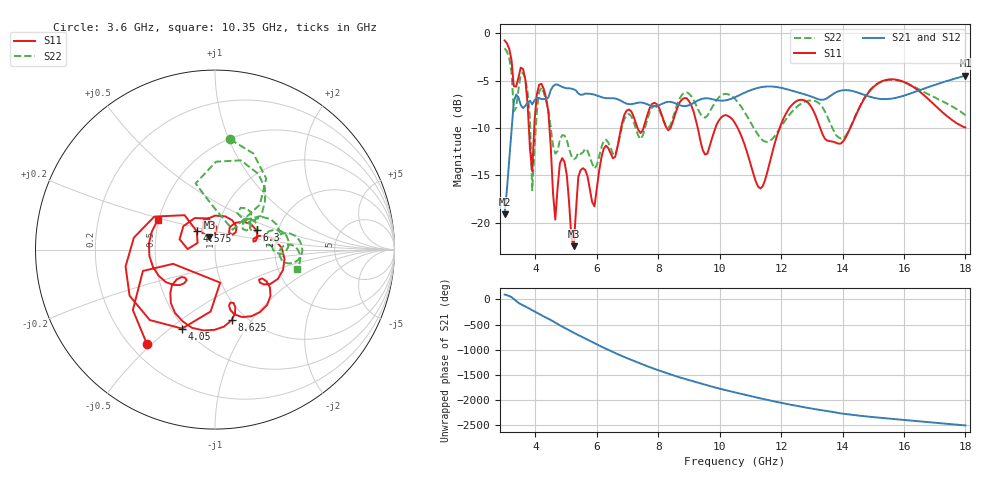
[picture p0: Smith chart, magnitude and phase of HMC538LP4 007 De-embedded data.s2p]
! Chelmsford, MA 01824
! http://www.hittite.com
! Tel: 978-250-3343
! Fax: 978-250-3373
! Device  :  HMC538LP4
! Description:  600 Analog Phase Shifter
! Frequency  :  6.0 GHz - 15.0 GHz
! Package  :  LP4  - 4x4 mm Quad Flatpack No-Lead (QFN) Plastic Package: 24 pin
! Ports  :  2 RF, 1 DC
!  Pin  3  = Rfin  = Port 1
!  Pin  16  = Rfout = Port 2
!  pin  21  = vCTL
! Voltages:  VCTL  = 0 to 5.0 Volts
! Currents :  Vb(V)  Vd(V)  Ib(mA)  Id(mA)
!  0.00  0.70  0.000000	0.484032
! Data:  The device was measured on evaluation board 111296-1.
!  Data was collected using a calibrated network analyzer.
!  The evaluation circuit board was modeled and simulated.This was use
!  to removed the evaluation board circuit from the measured data.
!  The reference plane is the center of the package pin.
! Misc:  Lot #
!Date Measured:  03 - 11 -2009
! Date:  03 - 17 -2009
! Note:
!  Hittite Microwave supplies this data as a sample of measured data at the
!  package pin for this package product.  Your particular data for this product
!  may vary.
!  Data was taken at 25 degrees C.
!  Hittite Microwave reserves the right to change this data at anytime.
# MHz S MA R 50
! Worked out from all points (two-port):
!   201 points, 3 GHz to 18 GHz, reference 50 ohm
!   highest |S21| = -4.46 dB at 18 GHz (marker M1); lowest = -19.1 dB at 3 GHz (marker M2)
!   |S21| within 3 dB of the highest: 3.909 GHz to 7.012 GHz (3.103 GHz wide, 56.8 % of centre); 9.097 GHz to end of sweep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
!   lowest |S11| = -22.5 dB at 5.25 GHz (marker M3), VSWR 1.16, Z = 46.6 + j6.4 ohm
!   |S11| at or under -10 dB: 4.461 GHz to 6.792 GHz (2.331 GHz wide, 41.4 % of centre); 10.59 GHz to 11.96 GHz (1.369 GHz wide, 12.1 % of centre); 13.27 GHz to 14.25 GHz (985.1 MHz wide, 7.16 % of centre)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
!   |S22| runs from -16.6 to -1.6 dB; largest |S21 - S12| = 0.0017
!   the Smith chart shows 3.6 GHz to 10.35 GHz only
!   S11 on the Smith chart (normalised r, x): 3.6 GHz: 0.27, -0.48; 4.05 GHz: 0.48, -0.55; 4.575 GHz: 0.80, +0.17; 6.3 GHz: 1.55, +0.36; 8.625 GHz: 0.85, -0.80; 10.35 GHz: 0.49, +0.19
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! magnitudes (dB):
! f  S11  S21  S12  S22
! 3 GHz  -0.8  -19.1  -19.1  -1.6
! 3.3 GHz  -5.6  -7.2  -7.2  -8.2
! 3.6 GHz  -3.8  -7.9  -7.9  -4.2
! 3.825 GHz  -12.2  -7.1  -7.1  -9.0
! 3.9 GHz  -14.6  -7.5  -7.5  -16.6
! 4.05 GHz  -6.4  -6.8  -6.8  -8.3
! 4.35 GHz  -6.8  -6.9  -6.9  -7.1
! 4.575 GHz  -16.9  -5.6  -5.6  -11.9
! 4.95 GHz  -13.6  -5.8  -5.8  -10.8
! 5.25 GHz  -22.5  -5.9  -5.9  -13.3
! 5.55 GHz  -14.3  -6.5  -6.5  -12.6
! 5.925 GHz  -18.3  -6.5  -6.5  -14.3
! 6.3 GHz  -11.9  -6.9  -6.9  -11.2
! 8.025 GHz  -7.8  -7.6  -7.6  -8.1
! 8.625 GHz  -7.9  -7.5  -7.5  -7.4
! 10.35 GHz  -8.9  -7.0  -7.0  -6.6
! 10.5 GHz  -9.5  -6.8  -6.8  -6.9
! 11.32 GHz  -16.4  -5.7  -5.7  -11.1
! 13.05 GHz  -8.2  -6.8  -6.8  -7.1
! 14.03 GHz  -11.4  -6.0  -6.0  -11.1
! 15.53 GHz  -4.9  -6.9  -6.9  -4.9
! 18 GHz  -9.9  -4.5  -4.5  -8.7
